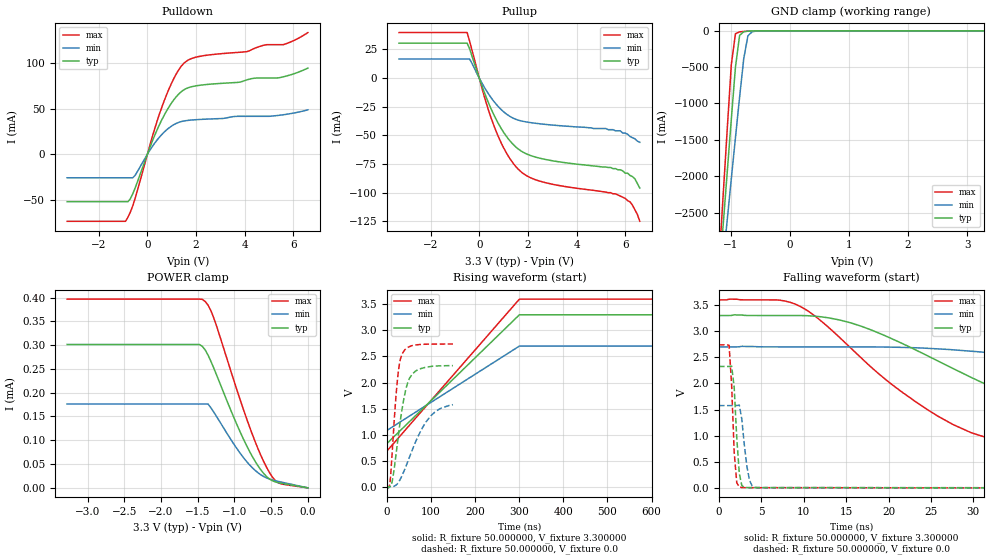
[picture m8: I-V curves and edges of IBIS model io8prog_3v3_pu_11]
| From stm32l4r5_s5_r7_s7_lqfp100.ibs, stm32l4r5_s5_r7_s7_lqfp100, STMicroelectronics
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|   Model io8prog_3v3_pu_11
[Model]  io8prog_3v3_pu_11
Model_type I/O
Polarity   Non-Inverting
Enable   Active-Low
Vinl =   0.990000V
Vinh =   2.310000V
Vmeas =  1.650000V
Cref =   100.000000nF
Rref =   1.000000k
Vref =   3.300000V
C_comp   2.267200pF   2.233100pF   2.322300pF
[Temperature Range]   25.000000   0.125000k   -40.000000
[Pullup Reference]   3.300000V   2.700000V   3.600000V
[Pulldown Reference]   0.0V   0.0V   0.0V
[POWER Clamp Reference]   3.300000V   2.700000V   3.600000V
[GND Clamp Reference]   0.0V   0.0V   0.0V
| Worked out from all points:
|   slope of the pulldown table from 0 to 0.495 V, typ, clamps not added: 15.3 ohm
|   slope of the pullup table from 0 to 0.495 V, typ, clamps not added: 18.1 ohm
|   GND clamp passes 1 mA (typ) near -0.58 V on its own axis
|   rising waveform, R_fixture 50.000000, V_fixture 3.300000: 20-80 % time 180ns typ, 180ns min, 180ns max; typ from 0.832 V to 3.3 V
|   rising waveform, R_fixture 50.000000, V_fixture 0.0: 20-80 % time 24.3ns typ, 50.8ns min, 14.6ns max; typ from 0.001 V to 2.33 V
|   falling waveform, R_fixture 50.000000, V_fixture 3.300000: 20-80 % time 21ns typ, 41.5ns min, 13.7ns max; typ from 3.3 V to 0.832 V
|   falling waveform, R_fixture 50.000000, V_fixture 0.0: 20-80 % time 499ps typ, 677ps min, 457ps max; typ from 2.33 V to 0.001 V
[Pulldown]
|Voltage   I(typ)   I(min)   I(max)
-3.3V     -51.86mA   -25.67mA   -73.32mA
-900mV    -51.86mA   -25.67mA   -73.32mA
-700mV    -48.68mA   -25.67mA   -63.27mA
-500mV    -36.68mA   -22.92mA   -47.9mA
200mV     14.09mA    8.363mA    18.97mA
700mV     43.2mA     24.54mA    59.15mA
1.2V      63.38mA    34mA       88.53mA
1.6V      72.01mA    36.89mA    101.8mA
4.1V      81.56mA    41.59mA    112.4mA
4.9V      83.55mA    41.59mA    120mA
5.6V      84.89mA    43.33mA    120.1mA
6.6V      94.39mA    48.68mA    133.3mA
[Pullup]
|Voltage   I(typ)   I(min)   I(max)
-3.3V     30.51mA    16.73mA    39.78mA
-500mV    30.51mA    16.73mA    39.78mA
-400mV    25.73mA    16.73mA    32.44mA
200mV     -11.99mA   -7.69mA    -15.6mA
500mV     -27.53mA   -17.49mA   -35.6mA
1V        -47.29mA   -29.37mA   -60.81mA
1.5V      -60.05mA   -35.95mA   -77.15mA
1.9V      -65.76mA   -38.13mA   -84.63mA
2.6V      -70.47mA   -40.14mA   -90.6mA
5.6V      -79mA      -46mA      -101mA
6.2V      -85mA      -51mA      -108mA
6.6V      -96mA      -56mA      -125mA
[GND_clamp]
|Voltage   I(typ)   I(min)   I(max)
-3.3V     -9.456A    -9.706A    -9.779A
-1.2V     -3.441A    -3.76A     -3.218A
-1.13V    -2.694A    -3.182A    -2.288A
-1.06V    -1.951A    -2.607A    -1.365A
-990mV    -1.216A    -2.035A    -464.9mA
-920mV    -500mA     -1.468A    -40.15mA
-850mV    -63.51mA   -913mA     -13.79mA
-780mV    -11.84mA   -384.3mA   -8.858mA
-710mV    -4.78mA    -70.26mA   -5.228mA
-640mV    -2.25mA    -14.29mA   -2.447mA
-430mV    -27.1uA    -149uA     -11.19uA
3.28V     0A         0A         0A
[POWER_clamp]
|Voltage   I(typ)   I(min)   I(max)
-3.28V    301.3uA    176.2uA    396.6uA
-1.48V    301.3uA    176.2uA    396.6uA
-1.4V     290uA      176.2uA    391.9uA
-1.36V    278.9uA    176.2uA    384uA
-1.28V    250.9uA    158.7uA    356.2uA
-1V       144.8uA    89.98uA    221.7uA
-840mV    90.38uA    56.36uA    147.8uA
-680mV    46.32uA    31.78uA    82.44uA
-560mV    23.38uA    20.73uA    42.33uA
-480mV    14.66uA    16.5uA     21.94uA
-400mV    10.77uA    13.43uA    10.23uA
0V        0A         0A         0A
[Ramp]
| variable   typ   min   max
dV/dt_r  1.39450/24.32029n   0.94482/54.54234n   1.64288/14.56534n
dV/dt_f  1.48066/21.06490n   0.97008/44.49579n   1.74725/13.65133n
R_load = 50.000000
[Rising Waveform]
R_fixture= 50.000000
V_fixture= 3.300000
V_fixture_min= 2.700000
V_fixture_max= 3.600000
|time   V(typ)   V(min)   V(max)
0s        832.2mV    1.083V     687.9mV
300.3ns   3.3V       2.7V       3.6V
600.6ns   3.3V       2.7V       3.6V
29.73us   3.3V       2.7V       3.6V
[Rising Waveform]
R_fixture= 50.000000
V_fixture= 0.0
V_fixture_min= 0.0
V_fixture_max= 0.0
|time   V(typ)   V(min)   V(max)
0s        929.1uV    1.395mV    658.7uV
6.907ns   5.861mV    4.453mV    94.66mV
12.61ns   142.3mV    5.769mV    767.7mV
22.52ns   757.8mV    49.89mV    1.951V
27.93ns   1.125V     113mV      2.345V
33.03ns   1.429V     196.1mV    2.518V
47.15ns   2.004V     485.7mV    2.673V
64.86ns   2.222V     863.5mV    2.721V
98.8ns    2.308V     1.357V     2.737V
149.5ns   2.325V     1.576V     2.739V
[Falling Waveform]
R_fixture= 50.000000
V_fixture= 3.300000
V_fixture_min= 2.700000
V_fixture_max= 3.600000
|time   V(typ)   V(min)   V(max)
0s        3.3V       2.7V       3.6V
9.61ns    3.3V       2.7V       3.473V
15.62ns   3.157V     2.7V       2.667V
24.62ns   2.527V     2.672V     1.495V
29.73ns   2.117V     2.617V     1.058V
33.63ns   1.831V     2.557V     907.2mV
46.55ns   1.158V     2.272V     764.1mV
60.06ns   970.6mV    1.923V     721.1mV
93.69ns   862.2mV    1.287V     693.7mV
149.5ns   832.2mV    1.083V     687.9mV
[Falling Waveform]
R_fixture= 50.000000
V_fixture= 0.0
V_fixture_min= 0.0
V_fixture_max= 0.0
|time   V(typ)   V(min)   V(max)
0s        2.325V     1.576V     2.739V
1.201ns   2.325V     1.576V     2.732V
1.502ns   2.333V     1.576V     1.969V
1.802ns   1.924V     1.576V     683.6mV
2.102ns   966.2mV    1.577V     99.05mV
2.402ns   279.8mV    1.586V     17.88mV
2.703ns   45.34mV    1.316V     6.39mV
3.604ns   5.102mV    151.6mV    4.383mV
4.505ns   4.666mV    6.472mV    4.371mV
149.5ns   929.1uV    1.395mV    658.7uV
